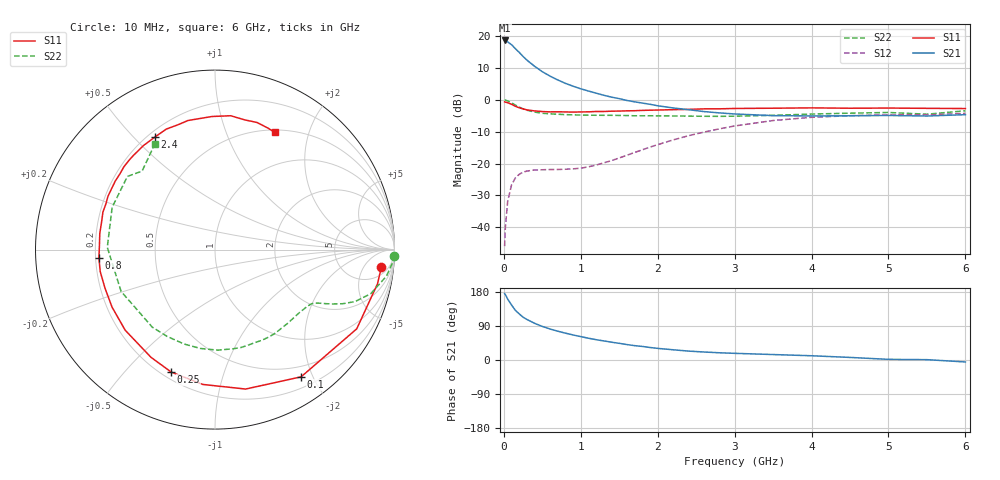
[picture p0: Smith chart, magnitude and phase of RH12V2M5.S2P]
! SIEMENS Small Signal Semiconductors
! BFR106
! Si NPN RF Bipolar Junction Transistor in SOT23
! VCE = 12 V  IC = 2.5 mA
! Common Emitter S-Parameters:  August  1996
# GHz  S  MA  R  50
!  f  S11  S21  S12  S22
! GHz  MAG  ANG  MAG  ANG  MAG  ANG  MAG  ANG
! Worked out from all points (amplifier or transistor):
!   36 points, 10 MHz to 6 GHz, reference 50 ohm
!   highest |S21| = 18.7 dB at 10 MHz (marker M1)
!   |S21| within 3 dB of that: start of sweep to 167.7 MHz
!   unconditionally stable (mu >= 1): 758.1 MHz to 1.821 GHz; 4.344 GHz to end of sweep
!   at 250 MHz: K = 0.35, MSG = 18.2 dB, |S12| = -22.7 dB
!   at 1.4 GHz: K = 1.21, MAG = 7.2 dB, |S12| = -19.1 dB
!   at 6 GHz: K = 1.02, MAG = -1.1 dB, |S12| = -4.2 dB
!   S11 on the Smith chart (normalised r, x): 10 MHz: 9, -13; 100 MHz: 0.35, -1.83; 250 MHz: 0.24, -0.68; 800 MHz: 0.21, -0.03; 2.4 GHz: 0.23, +0.58; 6 GHz: 0.53, +1.50
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0.01  0.9323 -6.0  8.642 175.4  0.005 88.8  0.9992 -1.9
0.02  0.9252 -11.9  8.536 172.4  0.01 83.5  0.9954 -3.7
0.05  0.9047 -29.2  8.214 160.7  0.0255 74.0  0.9667 -8.8
0.1  0.856 -55.9  7.415 145.2  0.046 61.2  0.9021 -15.8
0.15  0.7955 -77.6  6.42 131.2  0.0594 50.4  0.8316 -20.4
0.2  0.7543 -95.2  5.605 121.6  0.0676 44.2  0.7719 -23.0
0.25  0.7245 -109.7  4.847 113.0  0.0731 39.0  0.7221 -24.8
0.3  0.6981 -120.7  4.235 106.9  0.076 35.9  0.6901 -25.9
0.4  0.6724 -138.1  3.389 96.8  0.0791 32.4  0.6448 -27.5
0.5  0.6571 -150.8  2.785 88.6  0.0797 31.5  0.6178 -29.2
0.6  0.6494 -160.7  2.376 81.8  0.0804 32.5  0.6046 -31.3
0.8  0.6484 -175.9  1.827 70.9  0.0812 38.0  0.5881 -36.2
1.1  0.6501 166.5  1.381 57.5  0.0887 52.1  0.5767 -45.2
1.6  0.6744 145.4  0.982 40.7  0.1349 69.8  0.5686 -62.8
2.2  0.7035 124.5  0.749 27.0  0.2349 70.9  0.5605 -88.3
2.4  0.7109 118.1  0.703 23.5  0.2737 68.3  0.5567 -98.4
3  0.7348 101.8  0.602 17.6  0.3897 56.8  0.5556 -129.0
3.5  0.7418 91.3  0.567 14.4  0.4748 45.1  0.5727 -156.0
4.5  0.7414 77.0  0.564 6.8  0.5655 22.3  0.6197 157.6
5  0.7459 71.8  0.57 1.7  0.583 13.2  0.6358 140.1
5.5  0.7386 66.4  0.559 0.9  0.5833 8.6  0.597 132.9
6  0.7327 63.0  0.587 -5.2  0.6162 0.3  0.6759 119.8
